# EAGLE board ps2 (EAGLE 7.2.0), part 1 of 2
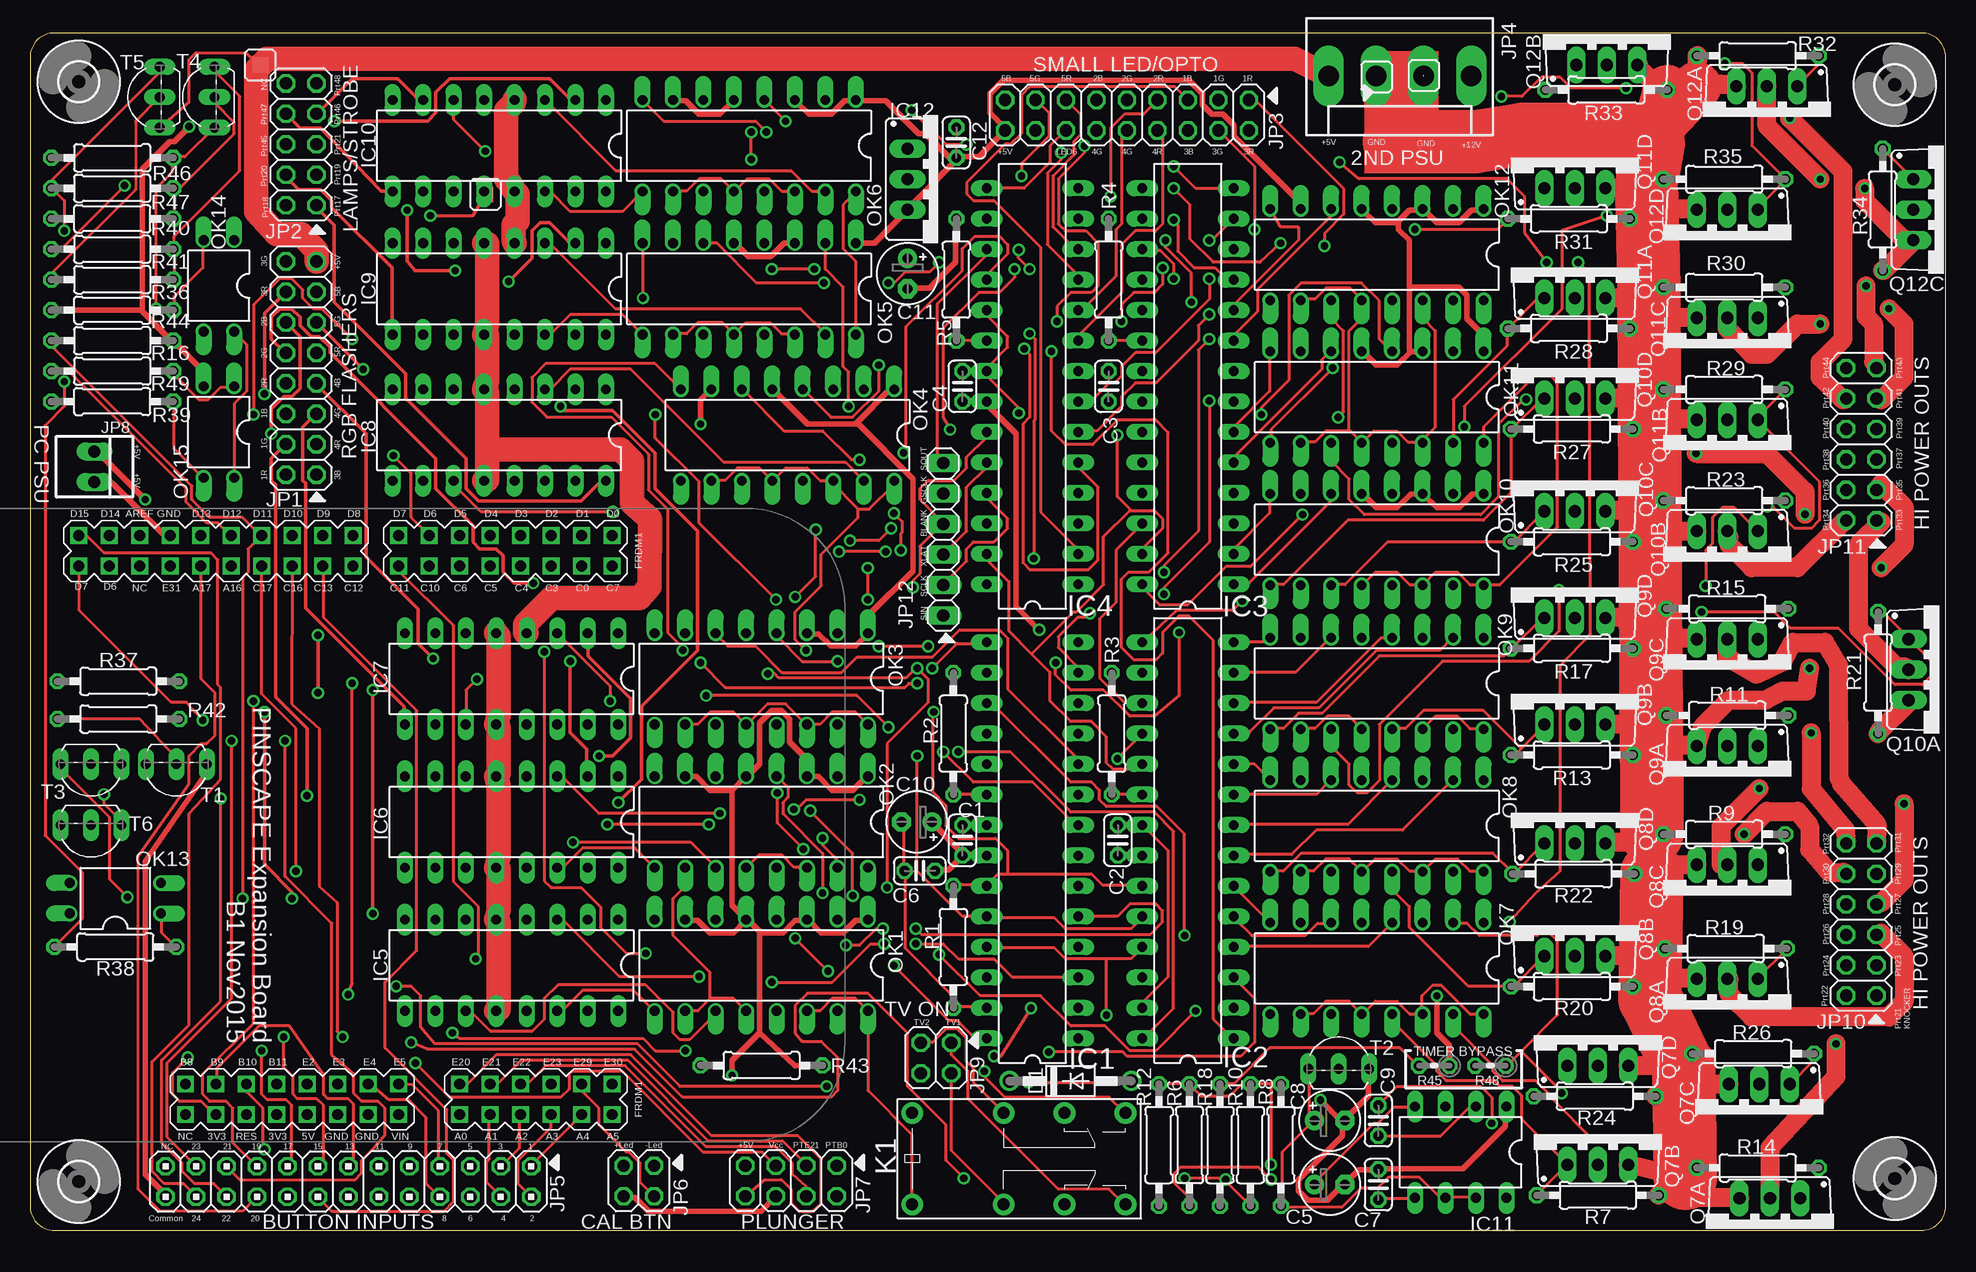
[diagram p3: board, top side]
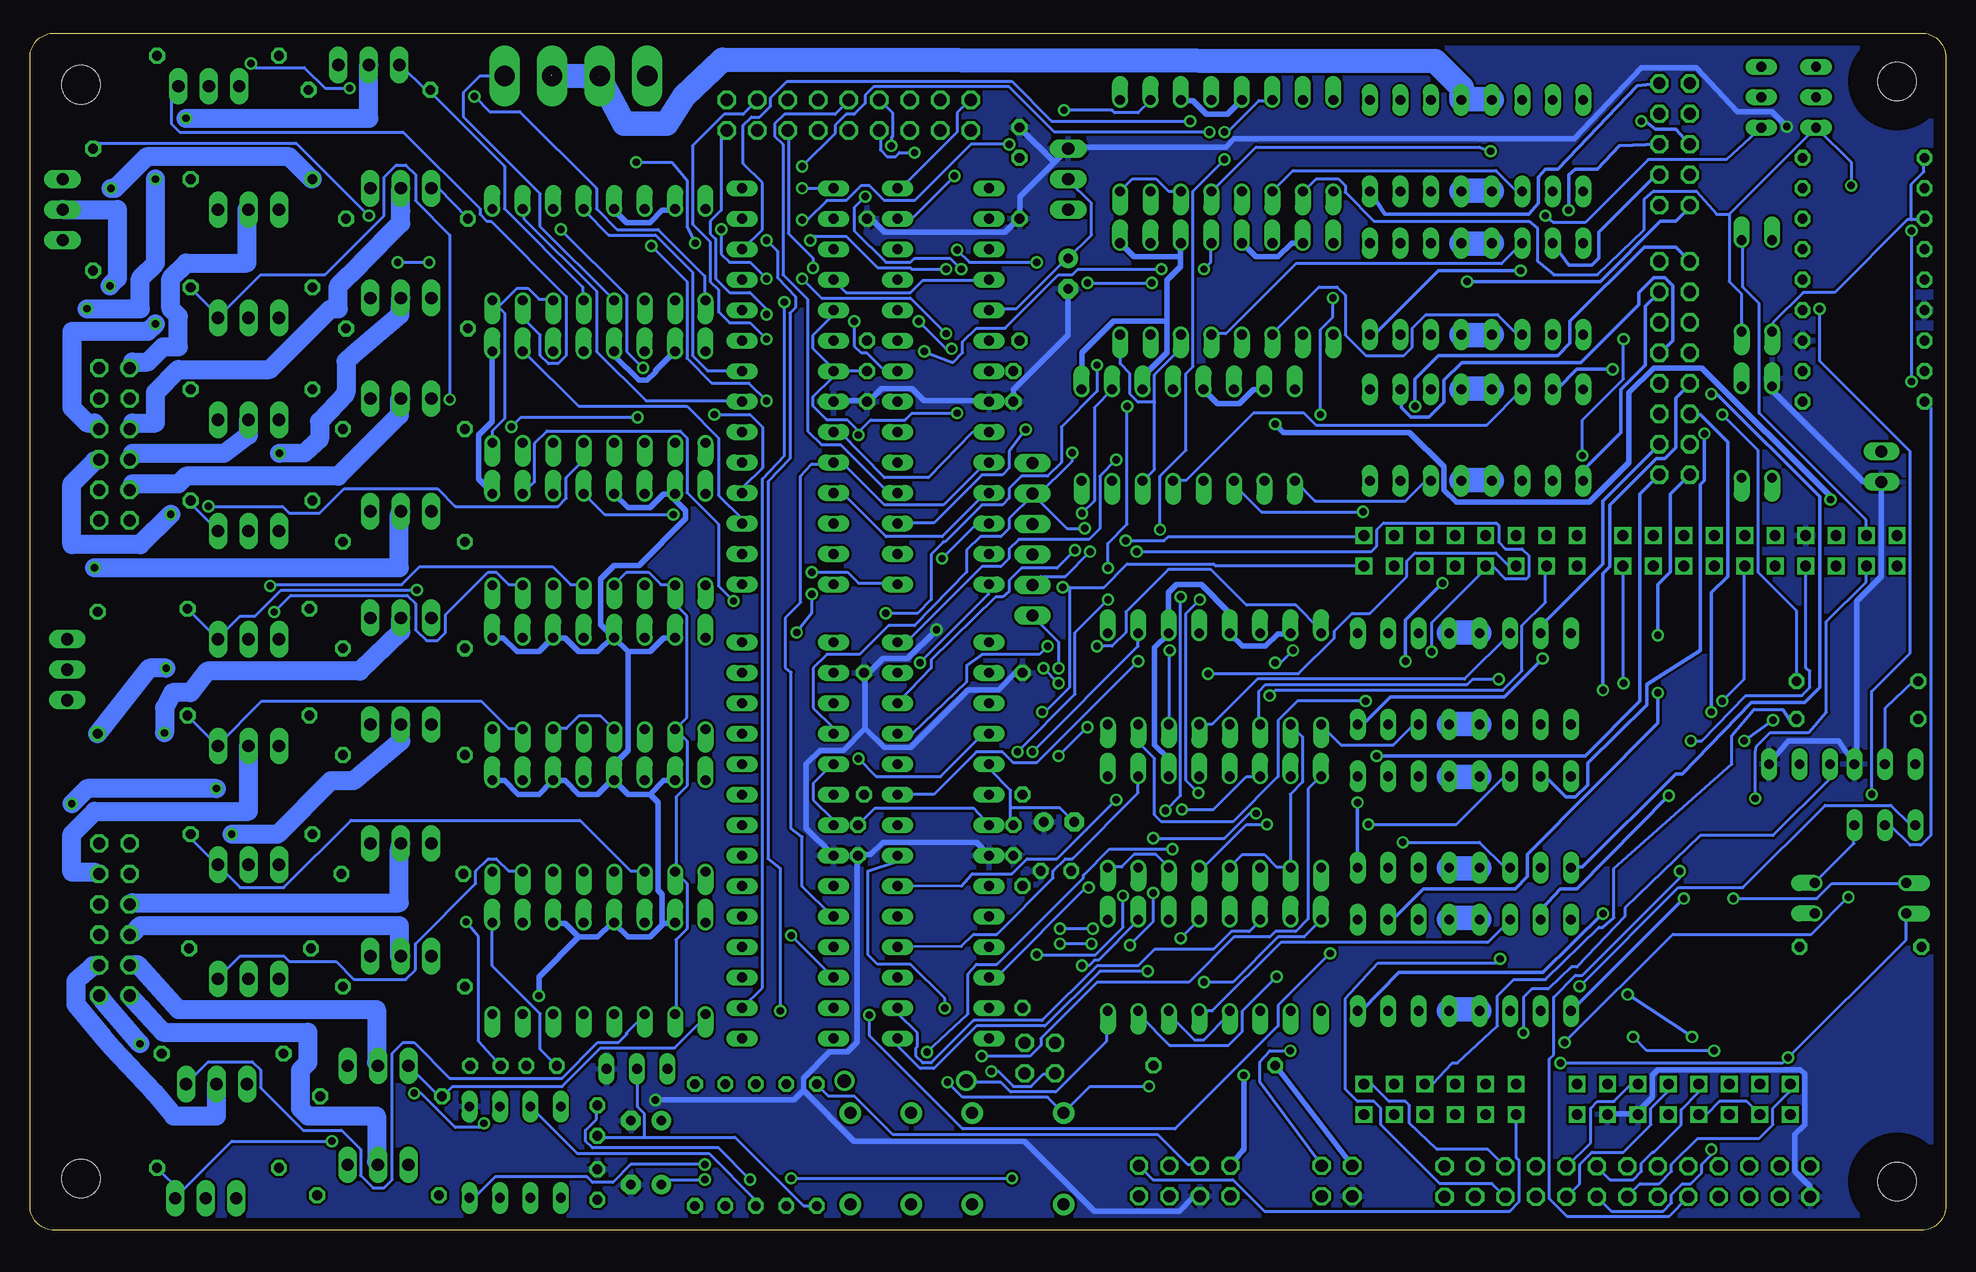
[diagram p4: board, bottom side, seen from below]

Size 159.69 x 99.81 mm. Coordinates in mm from the lower left corner, seen from the top.
Outline: 0,97.78 0,2.03 arc90 2.03,0 157.66,0 arc90 159.69,2.03 159.69,97.78 arc90 157.66,99.81 2.03,99.81 arc90 0,97.78
Copper layers (1*16): Top 0.035mm / dielectric 1.5mm / Bottom 0.035mm
Design rules "default": minimum track width 10mil, minimum drill 24mil, track to track 8mil, track to pad 8mil, pad to pad 8mil, via to via 8mil, smd to smd 8mil, copper to edge 40mil, drill to drill 8mil, minimum pad ring 10mil, minimum via ring 8mil, stop-mask expansion 4mil, vias tented up to drill 0mil, thermal gap 10mil
Net classes: 1 MOSFET Power & Ground: width 1.575 mm; 2 Lamps: width 0.305 mm; 3 Lamp Power & Ground: width 2.032 mm; 4 +5V: width 0.457 mm; 5 GND: width 0.457 mm

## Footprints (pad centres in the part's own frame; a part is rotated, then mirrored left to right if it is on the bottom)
C025-024X044 = drill 0.813 octagon: 1 -1.27,0; 2 1.27,0
E2,5-5 = drill 0.813 pad 1.6: + -1.27,0 | drill 0.813 pad 1.6 octagon: - 1.27,0
DO41-10 = drill 1.118: A 5.08,0; C -5.08,0
FRDM_KL25Z_NORMAL = drill 0.9 square: 3V3 24.13,-15.24; 5V 24.13,-7.62; A0 24.13,5.08; A1 24.13,7.62; A2 24.13,10.16; A3 24.13,12.7; A4 24.13,15.24; A5 24.13,17.78; AREF -24.13,-21.59; D0 -24.13,17.78; D1 -24.13,15.24; D2 -24.13,12.7; D3 -24.13,10.16; D4 -24.13,7.62; D5 -24.13,5.08; D6 -24.13,2.54; D7 -24.13,0; D8 -24.13,-3.81; D9 -24.13,-6.35; D10 -24.13,-8.89; D11 -24.13,-11.43; D12 -24.13,-13.97; D13 -24.13,-16.51; D14 -24.13,-24.13; D15 -24.13,-26.67; GND0 24.13,-2.54; GND1 24.13,-5.08; GND2 -24.13,-19.05; NC1 24.13,-17.78; NC2 -21.59,-21.59; P3V3 24.13,-10.16; PTA16 -21.59,-13.97; PTA17 -21.59,-16.51; PTB8 21.59,-17.78; PTB9 21.59,-15.24; PTB10 21.59,-12.7; PTB11 21.59,-10.16; PTC0 -21.59,15.24; PTC3 -21.59,12.7; PTC4 -21.59,10.16; PTC5 -21.59,7.62; PTC6 -21.59,5.08; PTC7 -21.59,17.78; PTC10 -21.59,2.54; PTC11 -21.59,0; PTC12 -21.59,-3.81; PTC13 -21.59,-6.35; PTC16 -21.59,-8.89; PTC17 -21.59,-11.43; PTD6 -21.59,-24.13; PTD7 -21.59,-26.67; PTE2 21.59,-7.62; PTE3 21.59,-5.08; PTE4 21.59,-2.54; PTE5 21.59,0; PTE20 21.59,5.08; PTE21 21.59,7.62; PTE22 21.59,10.16; PTE23 21.59,12.7; PTE29 21.59,15.24; PTE30 21.59,17.78; PTE31 -21.59,-19.05; RESET 24.13,-12.7; VIN 24.13,0
DIP28 = drill 0.813 long: 1 -15.24,-3.81; 2 -12.7,-3.81; 3 -10.16,-3.81; 4 -7.62,-3.81; 5 -5.08,-3.81; 6 -2.54,-3.81; 7 0,-3.81; 8 2.54,-3.81; 9 5.08,-3.81; 10 7.62,-3.81; 11 10.16,-3.81; 12 12.7,-3.81; 13 15.24,-3.81; 14 17.78,-3.81; 15 17.78,3.81; 16 15.24,3.81; 17 12.7,3.81; 18 10.16,3.81; 19 7.62,3.81; 20 5.08,3.81; 21 2.54,3.81; 22 0,3.81; 23 -2.54,3.81; 24 -5.08,3.81; 25 -7.62,3.81; 26 -10.16,3.81; 27 -12.7,3.81; 28 -15.24,3.81
DIL16 = drill 0.813 long: 1 -8.89,-3.81; 2 -6.35,-3.81; 3 -3.81,-3.81; 4 -1.27,-3.81; 5 1.27,-3.81; 6 3.81,-3.81; 7 6.35,-3.81; 8 8.89,-3.81; 9 8.89,3.81; 10 6.35,3.81; 11 3.81,3.81; 12 1.27,3.81; 13 -1.27,3.81; 14 -3.81,3.81; 15 -6.35,3.81; 16 -8.89,3.81
DIL08 = drill 0.813 long: 1 -3.81,-3.81; 2 -1.27,-3.81; 3 1.27,-3.81; 4 3.81,-3.81; 5 3.81,3.81; 6 1.27,3.81; 7 -1.27,3.81; 8 -3.81,3.81
TO220S = drill 1.016 long: 1 -2.54,-2.54; 2 0,-2.54; 3 2.54,-2.54
2X08 = drill 1.016 octagon: 1 -8.89,-1.27; 2 -8.89,1.27; 3 -6.35,-1.27; 4 -6.35,1.27; 5 -3.81,-1.27; 6 -3.81,1.27; 7 -1.27,-1.27; 8 -1.27,1.27; 9 1.27,-1.27; 10 1.27,1.27; 11 3.81,-1.27; 12 3.81,1.27; 13 6.35,-1.27; 14 6.35,1.27; 15 8.89,-1.27; 16 8.89,1.27
2X05 = drill 1.016 octagon: 1 -5.08,-1.27; 2 -5.08,1.27; 3 -2.54,-1.27; 4 -2.54,1.27; 5 0,-1.27; 6 0,1.27; 7 2.54,-1.27; 8 2.54,1.27; 9 5.08,-1.27; 10 5.08,1.27
2X09 = drill 1.016 octagon: 1 -10.16,-1.27; 2 -10.16,1.27; 3 -7.62,-1.27; 4 -7.62,1.27; 5 -5.08,-1.27; 6 -5.08,1.27; 7 -2.54,-1.27; 8 -2.54,1.27; 9 0,-1.27; 10 0,1.27; 11 2.54,-1.27; 12 2.54,1.27; 13 5.08,-1.27; 14 5.08,1.27; 15 7.62,-1.27; 16 7.62,1.27; 17 10.16,-1.27; 18 10.16,1.27
KK-156-4 = drill 1.7 pad 2.184 long: 1 -5.94,0; 2 -1.98,0; 3 1.98,0; 4 5.94,0
2X13 = drill 1.016 octagon: 1 -15.24,-1.27; 2 -15.24,1.27; 3 -12.7,-1.27; 4 -12.7,1.27; 5 -10.16,-1.27; 6 -10.16,1.27; 7 -7.62,-1.27; 8 -7.62,1.27; 9 -5.08,-1.27; 10 -5.08,1.27; 11 -2.54,-1.27; 12 -2.54,1.27; 13 0,-1.27; 14 0,1.27; 15 2.54,-1.27; 16 2.54,1.27; 17 5.08,-1.27; 18 5.08,1.27; 19 7.62,-1.27; 20 7.62,1.27; 21 10.16,-1.27; 22 10.16,1.27; 23 12.7,-1.27; 24 12.7,1.27; 25 15.24,-1.27; 26 15.24,1.27
2X02 = drill 1.016 octagon: 1 -1.27,-1.27; 2 -1.27,1.27; 3 1.27,-1.27; 4 1.27,1.27
2X04 = drill 1.016 octagon: 1 -3.81,-1.27; 2 -3.81,1.27; 3 -1.27,-1.27; 4 -1.27,1.27; 5 1.27,-1.27; 6 1.27,1.27; 7 3.81,-1.27; 8 3.81,1.27
22-23-2021 = drill 1 long: 1 -1.27,0; 2 1.27,0
2X06 = drill 1.016 octagon: 1 -6.35,-1.27; 2 -6.35,1.27; 3 -3.81,-1.27; 4 -3.81,1.27; 5 -1.27,-1.27; 6 -1.27,1.27; 7 1.27,-1.27; 8 1.27,1.27; 9 3.81,-1.27; 10 3.81,1.27; 11 6.35,-1.27; 12 6.35,1.27
1X06 = drill 1.016 long: 1 -6.35,0; 2 -3.81,0; 3 -1.27,0; 4 1.27,0; 5 3.81,0; 6 6.35,0
G5V-2 = drill 1 pad 1.8: 1 -8.89,-3.81; 4 -1.27,-3.81; 6 3.81,-3.81; 8 8.89,-3.81; 9 8.89,3.81; 11 3.81,3.81; 13 -1.27,3.81; 16 -8.89,3.81
DIL16' = drill 0.813 offset: 1 -8.89,-3.81; 2 -6.35,-3.81; 3 -3.81,-3.81; 4 -1.27,-3.81; 5 1.27,-3.81; 6 3.81,-3.81; 7 6.35,-3.81; 8 8.89,-3.81; 9 8.89,3.81; 10 6.35,3.81; 11 3.81,3.81; 12 1.27,3.81; 13 -1.27,3.81; 14 -3.81,3.81; 15 -6.35,3.81; 16 -8.89,3.81
DIL04 = drill 0.813 offset: 1 -1.27,-3.81; 2 1.27,-3.81; 3 1.27,3.81; 4 -1.27,3.81
TO220BV = drill 1.016 long: 1 -2.54,-2.54; 2 0,-2.54; 3 2.54,-2.54
0207/10 = drill 0.813 octagon: 1 -5.08,0; 2 5.08,0
0204V = drill 0.813 octagon: 1 -1.27,0; 2 1.27,0
TO92-EBC = drill 0.813 long: B 0,-1.27; C 2.54,-1.27; E -2.54,-1.27
JP0 = smd 1.27 x 1.27: P$1 0,1.27; P$2 0,1.27
3,2 = hole 3.2: 0,0

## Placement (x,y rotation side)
C1  100nF  [C025-024X044]  77.72,32.51 90 top
C2  100nF  [C025-024X044]  90.68,32.51 90 top
C3  100nF  [C025-024X044]  89.92,70.36 90 top
C4  100nF  [C025-024X044]  77.72,70.36 90 top
C5  1uF  [E2,5-5]  108.33,3.81 0 top
C6  4.7uF  [C025-024X044]  74.17,29.97 180 top
C7  100nF  [C025-024X044]  112.39,3.81 90 top
C8  1uF  [E2,5-5]  108.33,9.14 0 top
C9  100nF  [C025-024X044]  112.39,9.14 90 top
C10  100uF  [E2,5-5]  73.91,34.04 180 top
C11  100uF  [E2,5-5]  73.15,79.76 270 top
C12  100nF  [C025-024X044]  77.22,90.68 90 top
D1  1N4007  [DO41-10]  86.73,12.45 0 top
FRDM1  KL25Z  [FRDM_KL25Z_NORMAL]  30.73,33.78 270 top
IC1  TLC5940NT  [DIP28]  83.57,31.24 90 top
IC2  TLC5940NT  [DIP28]  96.52,31.24 90 top
IC3  TLC5940NT  [DIP28]  96.52,69.09 90 top
IC4  TLC5940NT  [DIP28]  83.57,69.09 90 top
IC5  ULN2064BN  [DIL16]  40.13,22.1 180 top
IC6  ULN2064BN  [DIL16]  40.13,34.04 180 top
IC7  ULN2064BN  [DIL16]  40.13,45.97 180 top
IC8  ULN2064BN  [DIL16]  39.12,66.29 180 top
IC9  ULN2064BN  [DIL16]  39.12,78.49 180 top
IC10  ULN2064BN  [DIL16]  39.12,90.42 180 top
IC11  ICM7555  [DIL08]  119.25,6.52 180 top
IC12  LD1117AV33  [TO220S]  75.69,87.63 270 top
JP1  M20-9760846  [2X08]  22.61,71.88 90 top
JP2  M20-9760546  [2X05]  22.61,90.54 90 top
JP3  M20-9760746  [2X09]  91.44,92.96 180 top
JP4  KK-156-4  [KK-156-4]  114.19,96.24 180 top
JP5  M20-9761346  [2X13]  26.54,4.06 180 top
JP6  M20-9760246  [2X02]  50.75,4.11 180 top
JP7  M20-9760446  [2X04]  63.44,4.11 180 top
JP8  22-23-2021  [22-23-2021]  5.37,63.67 270 top
JP9  M20-9760246  [2X02]  75.51,14.36 180 top
JP10  M20-9760646  [2X06]  152.65,25.91 90 top
JP11  M20-9760646  [2X06]  152.65,65.53 90 top
JP12  M20-9990646  [1X06]  76.12,57.61 90 top
K1  G5V-2  [G5V-2]  82.42,5.97 0 top
OK1  PC847  [DIL16']  60.96,22.1 180 top
OK2  PC847  [DIL16']  60.96,34.04 180 top
OK3  PC847  [DIL16']  60.96,45.97 180 top
OK4  PC847  [DIL16']  63.14,66.29 180 top
OK5  PC847  [DIL16']  59.94,78.49 180 top
OK6  PC847  [DIL16']  59.94,90.42 180 top
OK7  PC847  [DIL16']  112.27,21.84 180 top
OK8  PC847  [DIL16']  112.27,33.72 180 top
OK9  PC847  [DIL16']  112.27,45.59 180 top
OK10  PC847  [DIL16']  112.27,57.58 180 top
OK11  PC847  [DIL16']  112.27,69.46 180 top
OK12  PC847  [DIL16']  112.27,81.33 180 top
OK13  PC817  [DIL04]  7.11,27.69 90 top
OK14  PC817  [DIL04]  15.75,78.74 180 top
OK15  PC817  [DIL04]  15.75,66.55 180 top
Q7A  BUK7575-55A  [TO220BV]  145.03,0.13 180 top
Q7B  BUK7575-55A  [TO220BV]  130.68,8 0 top
Q7C  BUK7575-55A  [TO220BV]  144.15,9.65 180 top
Q7D  BUK7575-55A  [TO220BV]  130.68,16.26 0 top
Q8A  BUK7575-55A  [TO220BV]  141.48,18.41 180 top
Q8B  BUK7575-55A  [TO220BV]  128.78,25.4 0 top
Q8C  BUK7575-55A  [TO220BV]  141.48,27.94 180 top
Q8D  BUK7575-55A  [TO220BV]  128.78,34.8 0 top
Q9A  BUK7575-55A  [TO220BV]  141.48,37.85 180 top
Q9B  BUK7575-55A  [TO220BV]  128.78,44.7 0 top
Q9C  BUK7575-55A  [TO220BV]  141.48,46.74 180 top
Q9D  BUK7575-55A  [TO220BV]  128.78,53.59 0 top
Q10A  BUK7575-55A  [TO220BV]  159.13,46.74 270 top
Q10B  BUK7575-55A  [TO220BV]  141.48,55.75 180 top
Q10C  BUK7575-55A  [TO220BV]  128.78,62.48 0 top
Q10D  BUK7575-55A  [TO220BV]  128.78,71.88 0 top
Q11A  BUK7575-55A  [TO220BV]  128.78,80.26 0 top
Q11B  BUK7575-55A  [TO220BV]  141.48,65.02 180 top
Q11C  BUK7575-55A  [TO220BV]  141.48,73.53 180 top
Q11D  BUK7575-55A  [TO220BV]  128.78,89.41 0 top
Q12A  BUK7575-55A  [TO220BV]  144.78,92.84 180 top
Q12B  BUK7575-55A  [TO220BV]  131.44,99.69 0 top
Q12C  BUK7575-55A  [TO220BV]  159.51,85.09 270 top
Q12D  BUK7575-55A  [TO220BV]  141.48,82.55 180 top
R1  10K  [0207/10]  76.96,23.62 270 top
R2  4K  [0207/10]  76.96,41.4 90 top
R3  4K  [0207/10]  90.17,41.4 90 top
R4  4K  [0207/10]  89.92,79.25 90 top
R5  2.2K  [0207/10]  77.22,79.25 90 top
R6  1M  [0207/10]  96.65,7.11 90 top
R7  1K  [0207/10]  130.68,2.92 180 top
R8  2.2M  [0207/10]  104.27,7.11 270 top
R9  1K  [0207/10]  141.22,33.02 0 top
R10  100K  [0207/10]  101.73,7.11 270 top
R11  1K  [0207/10]  141.48,42.93 0 top
R12  100K  [0207/10]  94.11,7.11 270 top
R13  1K  [0207/10]  128.52,39.62 180 top
R14  1K  [0207/10]  144.02,5.21 0 top
R15  1K  [0207/10]  141.48,51.82 0 top
R16  10K  [0207/10]  6.86,74.17 180 top
R17  1K  [0207/10]  128.52,48.51 180 top
R18  47R  [0207/10]  99.19,7.11 270 top
R19  1K  [0207/10]  141.35,23.5 0 top
R20  1K  [0207/10]  128.52,20.32 180 top
R21  1K  [0207/10]  154.05,46.48 90 top
R22  1K  [0207/10]  128.65,29.72 180 top
R23  1K  [0207/10]  141.22,60.83 0 top
R24  1K  [0207/10]  130.43,11.18 180 top
R25  1K  [0207/10]  128.52,57.4 180 top
R26  1K  [0207/10]  143.64,14.73 0 top
R27  1K  [0207/10]  128.52,66.8 180 top
R28  1K  [0207/10]  128.27,75.18 180 top
R29  1K  [0207/10]  141.22,70.1 0 top
R30  1K  [0207/10]  141.22,78.61 0 top
R31  1K  [0207/10]  128.27,84.33 180 top
R32  1K  [0207/10]  144.02,97.92 0 top
R33  1K  [0207/10]  131.39,95.07 180 top
R34  1K  [0207/10]  154.43,85.09 90 top
R35  1K  [0207/10]  141.22,87.63 0 top
R36  560R  [0207/10]  6.86,76.71 0 top
R37  2.2K  [0207/10]  7.37,45.77 180 top
R38  220R  [0207/10]  7.11,23.62 0 top
R39  560R  [0207/10]  6.86,71.63 180 top
R40  10K  [0207/10]  6.86,84.33 0 top
R41  4.7K  [0207/10]  6.86,81.79 180 top
R42  2.2K  [0207/10]  7.37,42.62 180 top
R43  82R  [0207/10]  60.97,13.74 180 top
R44  4.7K  [0207/10]  6.86,79.25 180 top
R45  0R  [0204V]  117.04,13.72 180 top
R46  10K  [0207/10]  6.86,89.41 180 top
R47  22K  [0207/10]  6.86,86.87 180 top
R48  0R  [0204V]  121.73,13.72 180 top
R49  2.2K  [0207/10]  6.86,69.09 0 top
T1  2N4401  [TO92-EBC]  12.19,37.59 180 top
T2  2N4403  [TO92-EBC]  109.09,14.73 0 top
T3  2N4401  [TO92-EBC]  5.08,37.59 180 top
T4  2N4401  [TO92-EBC]  14.11,94.46 90 top
T5  2N4403  [TO92-EBC]  9.54,94.46 90 top
T6  2N4401  [TO92-EBC]  5.08,32.51 180 top
U$1  NETJUMPER  [JP0]  19.2,98.41 180 top
U$2  NETJUMPER  [JP0]  116.19,97.55 180 top
U$3  NETJUMPER  [JP0]  37.97,85.09 0 top
U$4  NETJUMPER  [JP0]  112.24,94.89 0 top
U$16  [3,2]  4.06,95.76 270 top
U$17  [3,2]  155.45,4.32 90 top
U$18  [3,2]  4.06,4.06 0 top
U$19  [3,2]  155.45,95.5 0 top

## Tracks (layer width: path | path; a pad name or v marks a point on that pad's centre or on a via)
3V3_KL25Z  (via drill 0.61)
  Top 0.254: v13.14,14.4 11.89,13.14 11.89,11.32 12.46,10.74 14.29,10.74 15.43,9.6 FRDM1.3V3 | 103.44,12.23 104.24,12.23 R8.1 | 103.44,12.23 101.73,12.23 R10.1 101.61,12.23 101.04,12.23 100.01,11.2 97.61,11.2 96.7,12.12 R6.2 96.58,12.23 94.18,12.23 R12.1 | 103.44,12.23 v103.44,5.49 | v32.12,13.95 34.98,11.09 44.23,11.09 44.92,11.77 44.92,13.03 45.15,13.26 49.38,13.26 56.12,6.51 61.04,6.51 JP7.5
  Bottom 0.254: OK13.4 3.31,26.4 3.31,24.23 v13.14,14.4 13.6,13.95 v32.12,13.95 | FRDM1.P3V3 20.57,9.72 19.89,9.72 18.86,10.74 16.57,10.74 15.54,9.72 FRDM1.3V3 | v103.44,5.49 109.61,5.49 111.1,4 112.81,4 113.27,4.46 120.93,4.46 122.64,2.74 122.99,2.74 IC11.8 | JP7.5 62.18,5.49 63.21,5.49 65.72,8 87.78,8 90.98,11.2 93.15,11.2 94.07,12.12 R12.1
+5V  (via drill 0.61)
  Top 0.457: OK10.5 111.1,61.38 112.24,60.24 113.96,60.24 115.1,61.38 116.01,61.38 OK10.3 116.24,61.27 117.27,60.24 119.1,60.24 120.24,61.38 121.16,61.38 OK10.1 | 115.1,73.27 OK11.3 | 115.1,73.27 113.96,72.12 112.24,72.12 111.1,73.27 OK11.5 | 113.96,84.01 114.99,85.04 116.01,85.04 OK12.3 116.24,85.04 117.27,84.01 119.1,84.01 120.13,85.04 121.16,85.04 OK12.1 | 113.96,84.01 112.13,84.01 OK12.5 | 114.99,78.64 114.99,82.53 114.07,83.44 114.07,83.9 113.96,84.01 | 114.99,78.64 114.99,73.38 115.1,73.27 | OK11.1 121.16,74.64 119.79,76.01 119.79,77.95 119.1,78.64 114.99,78.64 | v117.27,19.55 117.27,16.46 118.3,15.43 R45.1 | OK2.1 69.84,37.95 68.58,36.69 66.86,36.69 65.72,37.83 64.81,37.83 OK2.3 64.69,38.06 64.69,39.32 63.32,40.69 63.32,42.63 62.64,43.32 61.84,43.32 60.81,42.29 60.81,38.86 59.89,37.95 OK2.5 59.66,37.83 58.52,36.69 | OK3.3 64.81,49.72 65.72,49.72 66.75,48.69 68.81,48.69 69.84,49.72 OK3.1 69.95,49.95 69.95,51.32 73.61,54.98 73.61,62.64 68.92,67.32 | 58.52,36.69 56.69,36.69 55.55,37.83 54.63,37.83 OK2.7 | OK1.7 54.63,25.83 55.66,25.83 56.69,24.8 58.64,24.8 59.66,25.83 OK1.5 | 60.92,24.8 62.75,24.8 63.78,25.83 64.69,25.83 OK1.3 64.92,25.83 65.95,24.8 67.78,24.8 68.81,25.83 69.84,25.83 OK1.1 | 60.92,24.8 59.89,25.83 OK1.5 | 58.52,36.69 58.52,27.09 59.55,26.06 OK1.5 | v58.52,12.92 58.52,14.17 60.81,16.46 | 60.81,16.46 60.81,24.69 60.92,24.8 | OK5.3 62.87,82.3 61.72,81.15 59.89,81.15 58.75,82.3 OK5.5 | OK6.7 53.61,94.18 54.63,94.18 55.78,93.04 57.49,93.04 58.64,94.18 OK6.5 | OK6.3 63.78,94.18 64.92,93.04 66.75,93.04 67.89,94.18 68.81,94.18 OK6.1 69.04,94.18 71.32,94.18 74.07,91.44 74.64,91.44 76.81,89.27 C12.1
  Top 0.457: C12.1 77.27,89.5 79.1,89.5 81.27,91.67 JP3.18 81.27,91.9 80.01,93.15 80.01,94.75 81.15,95.9 96.58,95.9 97.73,94.75 97.73,93.84 98.53,93.04 99.44,93.04 100.36,92.13 100.36,91.21 105.84,85.72 105.84,85.15 OK12.7 | OK5.1 70.41,82.3 73.15,85.04 IC12.3 73.27,85.27 77.04,89.04 77.04,89.27 C12.1 | v9.6,60.92 5.6,64.92 5.37,64.92 JP8.1 | v55.89,67.21 55.89,69.27 56.69,70.07 OK4.7 | 68.92,67.32 68.81,67.21 64.81,67.21 61.95,70.07 OK4.5 | 68.92,67.32 71.67,70.07 72.01,70.07 OK4.1 | 60.81,16.46 63.78,13.72 R43.1
  Bottom 0.457: OK10.5 109.84,60.24 108.01,60.24 106.87,61.38 105.96,61.38 OK10.7 105.96,61.15 105.96,60.92 105.04,60.01 105.04,59.32 108.93,55.44 110.98,55.44 112.13,54.29 112.13,50.52 111.21,49.61 OK9.5 | OK11.1 121.16,67.44 122.3,66.29 122.3,62.64 121.16,61.49 OK10.1 | OK11.7 105.96,73.27 107.56,71.67 107.56,71.55 108.24,70.87 108.93,70.87 110.98,72.92 110.98,73.27 OK11.5 | OK12.7 105.96,85.04 106.98,85.04 108.01,84.01 109.96,84.01 110.98,85.04 OK12.5 | 106.87,25.6 105.96,25.6 OK7.7 | 106.87,25.6 108.01,24.46 109.84,24.46 110.98,25.6 OK7.5 111.21,25.6 112.36,24.46 113.96,24.46 | 113.96,24.46 115.1,25.6 116.01,25.6 OK7.3 | v117.27,19.55 117.27,21.14 113.96,24.46 | 108.01,36.35 106.87,37.49 105.96,37.49 OK8.7 | 108.01,36.35 109.84,36.35 110.98,37.49 OK8.5 | OK8.5 111.21,37.49 112.36,36.35 113.96,36.35 115.1,37.49 116.01,37.49 OK8.3 116.24,37.38 117.27,36.35 118.99,36.35 120.13,37.49 121.16,37.49 OK8.1 | 109.84,48.23 108.01,48.23 106.87,49.38 105.96,49.38 OK9.7 | 109.84,48.23 110.98,49.38 OK9.5 | OK9.5 111.21,49.38 112.36,48.23 113.96,48.23 115.1,49.38 116.01,49.38 OK9.3 116.24,49.26 117.27,48.23 119.1,48.23 120.24,49.38 121.16,49.38 OK9.1 | 109.84,48.23 109.84,40.01 110.87,38.98 110.87,37.72 OK8.5 | 108.01,36.35 107.33,35.66 107.33,28.35 106.98,28 106.98,25.72 106.87,25.6 | OK3.7 54.63,49.72 55.66,49.72 56.69,48.69 58.64,48.69 59.66,49.72 OK3.5 59.78,49.95 59.78,51.55 62.06,53.84 64.12,53.84 64.81,53.15 64.81,49.95 OK3.3 64.81,49.72 65.95,48.58 65.95,40.46 64.81,39.32 64.81,37.95 OK2.3 | JP7.7 59.55,5.49 58.64,6.63 58.52,6.74 v58.52,12.92 | OK5.7 54.52,82.3 55.66,81.15 57.49,81.15 58.64,82.3 OK5.5
  Bottom 0.457: 64.92,75.78 64.92,79.21 63.78,80.35 63.78,81.15 | 64.92,75.78 64.92,73.15 66.86,71.21 66.86,70.18 OK4.3 | 63.78,81.15 63.78,82.3 OK5.3 | 64.92,75.78 69.38,75.78 72.01,73.15 72.01,70.18 OK4.1 | OK6.3 63.66,94.18 62.75,94.18 61.61,93.04 59.89,93.04 58.75,94.18 OK6.5 | 63.78,81.15 67.67,81.15 68.81,82.3 OK5.1 | OK4.5 60.69,68.92 58.86,68.92 57.72,70.07 56.81,70.07 OK4.7 | v9.6,60.92 9.6,61.15 20.34,71.89 24.35,71.89 26.4,69.84 26.4,64.01 29.72,60.69 40.8,60.69 41.83,61.72 41.83,63.66 44.69,66.52 55.21,66.52 v55.89,67.21
+5V_PSU2  (via drill 0.61)
  Top 0.254: OK15.4 17.03,68.92 18.06,69.95 18.06,73.84 17.03,74.87 OK14.4 | v7.89,87.1 2.63,81.84 1.83,81.84 R41.2 | OK6.10 53.61,86.64 54.75,86.64 55.78,87.67 57.61,87.67 58.64,86.64 OK6.12 58.75,86.64 59.78,87.67 61.61,87.67 62.64,86.64 63.66,86.64 OK6.14 | OK5.16 68.81,74.75 68.81,80.81 67.78,81.84 67.78,85.5 68.81,86.53 OK6.16 | OK5.10 53.61,74.75 54.75,74.75 55.66,75.67 57.72,75.67 58.64,74.75 OK5.12 59.66,75.67 61.72,75.67 62.64,74.75 63.66,74.75 OK5.14 | OK4.10 56.81,62.52 57.95,62.52 58.98,63.55 60.81,63.55 OK4.12 61.95,62.52 62.98,63.55 64.81,63.55 65.84,62.52 66.86,62.52 OK4.14 66.75,62.41 69.04,60.12 | 69.04,60.12 69.95,60.12 72.01,62.18 72.01,62.41 OK4.16 | OK2.14 64.69,30.29 63.66,30.29 62.64,31.32 60.81,31.32 59.78,30.29 OK2.12 | OK3.10 54.63,42.18 55.66,42.18 56.69,43.2 58.64,43.2 59.66,42.18 OK3.12 59.78,42.18 61.49,43.89 62.98,43.89 64.69,42.18 OK3.14 64.81,42.18 65.84,42.18 66.86,43.2 68.81,43.2 OK3.16 | OK1.10 55.66,18.29 56.69,19.32 | 56.69,19.32 58.64,19.32 59.66,18.29 OK1.12 | OK1.14 65.84,18.29 66.86,19.32 68.81,19.32 69.84,18.29 OK1.16 69.84,18.17 69.84,11.66 73.5,8 73.5,2.17 K1.1 | 56.69,19.32 56.69,21.49 53.61,24.57 53.61,27.66 54.52,28.57 54.52,30.18 OK2.10 | 69.04,60.12 69.04,59.44 65.95,56.35 65.95,53.72 63.78,51.55 63.78,49.26 v64.69,48.35 | U$1.P$2 17.95,98.18 13.83,98.18 13.26,97.61 13.26,94.07 T5.E
  Bottom 0.254: v7.89,87.1 7.89,89.04 10.74,91.9 T5.E 10.86,91.9 18.06,84.7 | 18.06,84.7 18.06,79.1 17.03,78.07 17.03,74.98 OK14.4 | OK6.16 67.78,87.67 65.84,87.67 64.81,86.64 63.78,86.64 OK6.14 | 65.95,69.04 65.95,63.44 66.86,62.52 OK4.14 | 65.95,69.04 65.95,71.32 63.78,73.5 63.78,74.64 OK5.14 | 65.95,69.04 67.32,69.04 68.01,69.72 68.01,71.44 68.81,72.24 68.81,74.64 OK5.16 | OK2.12 59.66,30.29 58.64,31.32 56.81,31.32 55.78,30.29 54.63,30.29 OK2.10 54.63,30.4 54.63,36.35 53.61,37.38 53.61,41.15 54.52,42.06 OK3.10 | OK2.16 69.84,30.29 68.69,30.29 67.67,31.32 65.84,31.32 64.81,30.29 OK2.14 | D1.C 81.61,12.34 78.75,12.34 77.95,11.54 74.18,11.54 69.95,15.77 69.95,18.29 OK1.16 | OK1.12 59.78,18.29 59.78,17.95 61.84,15.89 62.64,15.89 64.69,17.95 64.69,18.29 OK1.14 | v64.69,48.35 64.69,42.18 OK3.14 | 18.06,84.7 19.09,84.7 20.8,86.64 24.35,86.64 25.15,85.95 25.15,83.44 29.03,79.67 32.69,79.67 34.06,80.81 34.06,83.55 34.75,84.12 47.66,84.12 50.06,86.53 50.06,87.1 50.63,87.67 52.46,87.67 53.49,86.64 OK6.10
+12V
  Top 0.254: OK12.10 105.96,77.61 107.1,77.61 108.01,78.52 110.07,78.52 110.98,77.61 OK12.12 110.98,77.5 110.98,76.01 109.96,74.98 109.96,66.64 | 109.96,66.64 110.07,66.64 110.98,65.72 OK11.12 111.1,65.72 112.01,66.64 113.96,66.64 114.87,65.72 116.01,65.72 OK11.14 116.01,65.84 117.16,66.98 117.16,74.98 116.13,76.01 116.13,77.5 OK12.14 | 109.96,66.64 108.01,66.64 107.1,65.72 105.96,65.72 OK11.10 | OK7.10 105.96,18.06 106.98,18.06 108.01,19.09 109.96,19.09 110.98,18.06 OK7.12 111.1,18.06 112.13,19.09 113.96,19.09 114.99,18.06 116.01,18.06 OK7.14 116.01,18.17 116.01,19.55 116.93,20.46 117.61,20.46 120.02,18.06 121.16,18.06 OK7.16 | OK10.12 111.1,53.84 112.13,54.86 113.96,54.86 114.99,53.84 116.01,53.84 OK10.14 116.13,53.84 117.16,54.86 118.99,54.86 120.02,53.84 121.16,53.84 OK10.16 121.27,53.84 122.53,53.84 127.33,58.64 127.33,70.64 126.76,71.21 125.39,71.21 121.16,66.98 OK11.16 | OK8.10 105.96,29.95 106.98,29.95 108.01,30.98 109.96,30.98 110.98,29.95 OK8.12 111.1,29.95 112.13,30.98 113.96,30.98 114.99,29.95 116.01,29.95 OK8.14 116.13,29.95 117.16,30.98 118.99,30.98 120.02,29.95 121.16,29.95 OK8.16 | OK9.10 105.96,41.83 107.1,41.83 108.13,42.86 109.96,42.86 110.98,41.83 OK9.12 | OK9.14 117.16,42.86 118.99,42.86 120.02,41.83 121.16,41.83 OK9.16
  Bottom 0.254: OK11.16 121.16,66.64 120.13,67.67 120.13,76.47 121.16,77.5 OK12.16 120.59,77.04 119.1,78.52 118.19,78.52 117.27,77.61 116.13,77.61 OK12.14 | JP4.1 122.19,96.24 123.56,94.87 123.56,92.81 117.16,86.41 117.16,83.67 111.1,77.61 OK12.12 | OK10.12 110.98,53.84 109.96,54.86 108.13,54.86 107.1,53.84 105.96,53.84 OK10.10 105.84,53.72 105.84,52.12 104.93,51.21 104.93,42.75 105.84,41.83 OK9.10 105.84,41.72 104.93,40.8 104.93,37.03 105.84,36.12 105.84,29.95 OK8.10 104.93,28.92 104.93,25.15 105.84,24.23 105.84,18.06 OK7.10 | OK9.14 116.01,41.83 114.99,41.83 113.96,42.86 112.13,42.86 111.1,41.83 OK9.12
ALT_MOSFETIN1  (via drill 0.61)
  Top 0.254: v123.33,25.72 125.5,28.12 127.56,29.95 127.56,47.09 130.07,49.72 129.96,74.3 129.96,79.78 v129.04,80.7 | v126.42,80.7 124.59,83.1 124.59,86.18 123.1,87.67 110.76,87.67 v109.16,89.04 | v104.24,82.3 102.53,80.7 98.64,80.7 96.7,82.64 96.7,85.5 v95.33,86.87
  Bottom 0.254: R48.2 122.3,15.77 122.3,24.46 v123.33,25.72 | v129.04,80.7 v126.42,80.7 | v109.16,89.04 106.19,89.04 104.93,87.55 104.93,83.67 v104.24,82.3 | v95.33,86.87 IC3.15
DARLINGTONIN1  (via drill 0.61)
  Top 0.254: IC1.28 78.75,16 77.27,17.49 76.58,17.49 v72.01,22.06
  Bottom 0.254: v72.01,22.06 71.44,22.06 70.98,22.52 70.64,22.52 67.32,25.83 OK1.2
DARLINGTONIN2  (via drill 0.61)
  Top 0.254: v63.78,24.35 v66.52,21.6
  Bottom 0.254: v66.52,21.6 70.52,21.6 75.09,17.03 80.81,17.03 84.35,13.49 85.5,13.49 87.33,15.32 87.33,16 IC1.1 | v63.78,24.35 62.29,25.83 OK1.4
DARLINGTONIN3
  Bottom 0.254: IC1.2 87.33,18.52 87.33,18.06 85.72,16.46 85.72,15.32 85.84,15.2 85.84,14.52 85.27,13.95 84.58,13.95 81.04,17.49 75.32,17.49 70.75,22.06 67.32,22.06 65.95,23.43 61.04,23.43 59.55,24.92 58.06,24.92 57.15,25.83 OK1.6
DARLINGTONIN4  (via drill 0.61)
  Top 0.254: v73.84,23.89 76.12,23.89 77.38,22.63 80.35,22.63 81.84,21.14 87.33,21.14 IC1.3 | v71.21,23.89 70.07,23.89 66.86,20.69 v61.84,20.69
  Bottom 0.254: v71.21,23.89 v73.84,23.89 | v61.84,20.69 59.44,20.69 55.66,24.46 53.49,24.46 52.12,25.83 OK1.8
DARLINGTONIN5
  Bottom 0.254: OK2.2 67.32,37.83 67.32,36.46 72.81,30.98 73.38,30.98 74.41,29.95 74.41,29.38 79.1,24.69 81.04,24.69 82.07,23.66 IC1.4
DARLINGTONIN6  (via drill 0.61)
  Top 0.254: v73.84,25.15 74.3,24.69 93.38,24.69 94.41,25.72 94.41,26.63 93.84,27.2 91.67,27.2 90.64,26.18 87.44,26.18 IC1.5 | v71.09,25.15 70.52,25.15 69.15,23.77 v68.01,23.77 | v66.06,28.12 66.06,31.43 62.75,34.75 62.75,35.66 63.21,36.12 63.21,36.92 62.29,37.83 OK2.4
  Bottom 0.254: v71.09,25.15 v73.84,25.15 | v68.01,23.77 66.06,25.72 v66.06,28.12
DARLINGTONIN7  (via drill 0.61)
  Top 0.254: v63.66,35.09 63.89,35.09 64.69,35.89 v69.15,35.89
  Bottom 0.254: v63.66,35.09 61.04,35.09 58.29,37.83 57.15,37.83 OK2.6 | v69.15,35.89 74.07,30.98 76.58,30.98 77.84,29.72 81.15,29.72 82.07,28.69 IC1.6
DARLINGTONIN8  (via drill 0.61)
  Top 0.254: v80.35,14.52 80.92,14.52 v83.44,18.52
  Bottom 0.254: v83.44,18.52 83.44,19.32 86.3,22.17 89.04,22.17 89.84,22.97 89.84,29.95 87.44,30.75 87.44,31.2 IC1.7 | v80.35,14.52 76.35,14.52 75.44,15.43 75.44,16 70.75,20.69 63.09,20.69 59.32,24.46 56.35,24.46 55.89,24.92 54.18,24.92 53.15,25.95 53.15,36.8 52.12,37.83 OK2.8
DARLINGTONIN9  (via drill 0.61)
  Top 0.254: v76.12,39.89 78.64,37.38 83.55,37.38 87.1,33.83 87.33,33.83 IC1.8
  Bottom 0.254: v76.12,39.89 67.32,48.69 67.32,49.72 OK3.2
DARLINGTONIN10  (via drill 0.61)
  Top 0.254: v67.32,47.43 64.35,47.43 62.29,49.49 62.29,49.72 OK3.4
  Bottom 0.254: v67.32,47.43 75.78,38.98 77.72,38.98 78.64,39.89 80.81,39.89 84.35,36.35 87.33,36.35 IC1.9
DARLINGTONIN11
  Top 0.254: IC1.10 87.33,38.86 87.33,39.32 81.5,45.15 81.5,49.38 80.81,50.06 77.5,50.06 75.21,47.78 68.92,47.78 67.67,46.52 62.64,46.52 60.47,48.69 58.18,48.69 57.15,49.72 OK3.6
DARLINGTONIN12  (via drill 0.61)
  Top 0.254: v70.75,48.69 v74.87,48.69
  Bottom 0.254: v74.87,48.69 75.55,48.01 80.35,48.01 81.61,47.09 81.61,45.72 86.18,41.38 IC1.11 | v70.75,48.69 69.49,48.69 68.35,49.84 68.35,51.55 64.81,55.09 61.27,55.09 58.29,52.12 54.18,52.12 52.12,50.06 52.12,49.84 OK3.8
DARLINGTONIN13  (via drill 0.61)
  Top 0.254: v72.58,56.69 72.58,58.06 72.69,58.18 72.69,59.09 v72.01,59.78
  Bottom 0.254: v72.58,56.69 74.07,55.21 77.04,55.21 78.07,54.18 78.07,53.26 78.64,52.81 79.21,52.81 84.58,47.55 84.58,46.86 87.33,44.01 IC1.12 | v72.01,59.78 70.98,60.81 70.98,68.58 69.49,70.07 OK4.2
DARLINGTONIN14  (via drill 0.61)
  Top 0.254: v88.35,51.44 88.01,51.09 87.33,51.09 85.72,49.49 85.72,48.58 87.33,46.98 87.33,46.52 IC1.13 | v70.75,72.12 70.75,69.95 68.58,67.78 66.75,67.78 64.47,70.07 OK4.4
  Bottom 0.254: v88.35,51.44 85.72,51.44 84.58,52.58 84.58,56.35 83.55,57.38 83.44,57.38 80.35,60.47 78.64,60.47 78.07,61.04 78.07,61.84 77.04,62.87 74.87,62.87 73.72,64.01 73.72,66.98 70.75,69.95 v70.75,72.12
DARLINGTONIN15  (via drill 0.61)
  Top 0.254: v69.15,64.24 68.47,64.24 66.06,66.64 62.87,66.64 59.44,70.07 OK4.6
  Bottom 0.254: v69.15,64.24 70.52,62.87 70.52,58.52 71.44,57.61 77.27,57.61 78.07,56.81 78.07,56.01 78.75,55.32 80.35,55.32 86.64,49.03 87.33,49.03 IC1.14
DARLINGTONIN16  (via drill 0.61)
  Top 0.254: v75.21,46.86 77.27,48.92 79.67,48.92 IC1.15 | v73.95,45.61 73.27,45.61 72.92,45.26 57.95,45.26 v55.89,47.32 | v54.41,48.35 54.41,48.58 53.15,49.84 53.15,60.12 51.55,61.72 51.55,64.69 48.46,67.78 43.09,67.78 41.83,69.04 41.83,71.09 42.98,72.24 52.12,72.24 OK4.8
  Bottom 0.254: v73.95,45.61 v75.21,46.86 | v55.89,47.32 55.44,47.32 v54.41,48.35
DARLINGTONIN17  (via drill 0.61)
  Top 0.254: OK5.2 66.29,80.12 67.78,78.64 67.78,72.01 68.24,71.55 v68.24,68.69 | v69.84,52.58 v69.84,55.21 | v77.38,39.89 81.72,39.89 86.75,34.86 93.73,34.86 95.33,33.26 95.33,18.52 92.81,16 IC2.28
  Bottom 0.254: v68.24,68.69 68.24,58.86 69.84,57.26 v69.84,55.21 | v69.84,52.58 72.58,49.84 72.58,44.69 v77.38,39.89
DARLINGTONIN18  (via drill 0.61)
  Top 0.254: v65.38,80.12 v61.84,80.12 | v85.15,73.27 85.15,66.64 86.3,65.49 88.58,65.49 90.64,67.55 93.84,67.55 94.87,66.52 94.87,56.46 93.27,54.86 91.55,54.86 90.98,54.29 90.98,48.58 92.01,47.55 93.84,47.55 94.41,48.12 94.41,49.84 95.78,51.21 96.58,51.21 98.64,49.15 98.64,17.6 100.24,16 IC2.1
  Bottom 0.254: v61.84,80.12 61.27,80.7 61.27,82.3 OK5.4 | v65.38,80.12 72.35,80.12 72.81,79.67 73.95,79.67 78.41,75.21 80.81,75.21 81.95,74.07 81.95,73.15 82.75,72.35 v85.15,73.27
DARLINGTONIN19  (via drill 0.61)
  Top 0.254: OK5.6 57.26,82.3 60.58,78.98 v66.18,78.98 | v71.55,78.98 72.01,78.98 72.92,79.9 74.98,79.9 v75.78,80.7 | v82.41,81.72 82.41,81.04 v83.33,80.12 | v94.64,82.53 94.64,81.95 96.81,79.78 v96.81,77.38
  Bottom 0.254: v71.55,78.98 v66.18,78.98 | v75.78,80.7 81.38,80.7 v82.41,81.72 | v83.33,80.12 86.18,80.12 86.3,80.24 89.04,80.24 91.67,82.87 94.3,82.87 v94.64,82.53 | v96.81,77.38 96.81,64.58 98.64,62.64 98.64,20.23 IC2.2
DARLINGTONIN20  (via drill 0.61)
  Top 0.254: v51.09,77.72 51.09,82.3 OK5.8 | v52.12,68.01 52.12,66.06 55.78,62.41 55.78,58.98 v62.18,52.58 | v62.29,36.46 62.29,33.95 v64.47,31.77 | v84.92,14.86 91.1,14.86 91.44,14.52 100.93,14.52 102.07,15.66 102.07,19.32 100.36,21.03 IC2.3
  Bottom 0.254: v51.09,77.72 51.09,76.12 52.12,75.09 v52.12,68.01 | v62.18,52.58 63.32,51.44 63.32,37.49 v62.29,36.46 | v64.47,31.77 69.72,31.77 71.89,29.6 71.89,29.38 79.1,22.17 80.81,22.17 81.5,21.37 81.5,18.06 v84.92,14.86
DARLINGTONIN21  (via drill 0.61)
  Top 0.254: v95.33,84.24 95.67,83.78 95.67,81.61 97.04,80.24 98.75,80.24 99.78,79.21 IC3.11 | v78.07,90.53 76.35,90.53 v73.5,93.38
  Bottom 0.254: v95.33,84.24 94.87,84.24 93.27,85.84 91.67,85.84 90.41,87.1 89.72,87.1 88.47,85.84 85.95,85.84 81.27,90.53 v78.07,90.53 | v73.5,93.38 69.49,93.38 69.27,93.15 67.32,93.15 66.29,94.18 OK6.2
DARLINGTONIN22  (via drill 0.61)
  Top 0.254: v62.98,92.47 OK6.4
  Bottom 0.254: v62.98,92.47 74.52,92.47 77.84,95.78 96.58,95.78 97.95,94.41 97.95,93.73 98.87,92.81 99.56,92.81 100.24,92.13 100.24,88.92 98.64,87.33 98.64,83.44 100.24,81.84 IC3.12
DARLINGTONIN23  (via drill 0.61)
  Top 0.254: v60.12,89.27 v60.12,91.55 | v65.49,58.41 65.49,54.52 v63.78,52.81 | v65.04,34.98 68.58,31.43 v68.58,27.89 | v75.78,22.97 79.21,19.55 84.24,19.55 86.75,17.03 89.61,17.03 91.67,14.97 93.84,14.97 v97.16,18.29 | v98.3,82.53 98.53,82.53 IC3.13
  Bottom 0.254: v60.12,91.55 59.89,91.55 57.26,94.18 56.24,94.18 OK6.6 | v60.12,89.27 62.75,86.64 62.75,72.01 63.32,71.44 63.32,65.04 65.49,62.87 v65.49,58.41 | v63.78,52.81 63.78,36.23 v65.04,34.98 | v68.58,27.89 68.58,25.26 70.87,22.97 v75.78,22.97 | v97.16,18.29 97.16,30.18 98.18,30.98 98.18,62.41 96.36,64.35 96.36,76.47 95.9,76.92 95.9,77.84 97.38,79.44 97.38,81.61 v98.3,82.53
DARLINGTONIN24  (via drill 0.61)
  Top 0.254: IC3.14 97.16,86.87 v95.33,88.7 | v61.38,91.55 60.47,92.47 52.81,92.47 51.09,94.18 OK6.8
  Bottom 0.254: v95.33,88.7 92.58,91.44 92.58,92.13 91.67,93.04 90.98,93.04 90.07,93.95 90.07,94.64 89.38,95.33 78.07,95.33 74.3,91.55 v61.38,91.55
DARLINGTONOUT1  (via drill 0.61)
  Top 0.305: v24,49.61 v24,44.81
  Bottom 0.305: v24,44.81 24,42.29 34.86,31.32 34.86,29.49 35.89,28.46 43.55,28.46 46.06,25.95 46.41,25.95 IC5.2 | v24,49.61 24,53.84 22.97,54.86 22.97,61.38 21.37,62.98 JP1.2
DARLINGTONOUT2  (via drill 0.61)
  Top 0.305: v23.09,36.23 23.09,41.83 20.46,44.46 20.46,62.18 20.12,62.52 20.12,64.35 21.26,65.49 JP1.4
  Bottom 0.305: v23.09,36.23 30.75,28.46 32.12,28.46 33.72,26.75 33.72,25.95 IC5.7
DARLINGTONOUT3  (via drill 0.61)
  Top 0.305: v21.83,27.66 21.83,28.23 19.55,30.52 v19.55,43.2
  Bottom 0.305: v21.83,27.66 31.2,18.29 IC5.9 | v19.55,43.2 19.55,53.15 18.17,54.52 18.17,65.72 20.46,68.01 21.26,68.01 JP1.6
DARLINGTONOUT4  (via drill 0.61)
  Top 0.305: v28.57,45.03 v28.57,26.4
  Bottom 0.305: IC5.16 48.69,18.29 45.61,21.49 33.6,21.49 v28.57,26.4 | v28.57,45.03 28.57,54.75 28,55.32 28,60.47 24.12,64.35 23.43,64.35 22.52,65.27 22.52,69.38 21.37,70.52 JP1.8
DARLINGTONOUT5  (via drill 0.61)
  Top 0.305: v45.03,47.43 45.03,41.49 46.41,40.12 46.41,37.95 IC6.2 | v41.95,53.95 40.35,53.95 39.43,54.86 39.43,56.24 38.86,56.81 37.49,56.81 36.92,57.38 36.92,58.75 33.83,61.84 33.83,64.35 25.03,73.15 25.03,73.61 24.12,74.52 23.43,74.52 22.52,75.44 22.52,76.12 21.83,76.81 20.8,76.81 20.12,76.12 20.12,74.3 21.26,73.15 JP1.10
  Bottom 0.305: v45.03,47.43 45.03,50.86 v41.95,53.95
DARLINGTONOUT6  (via drill 0.61)
  Top 0.305: v20.12,66.41 20.12,68.47 21.14,69.49 21.83,69.49 22.52,70.18 22.52,74.52 21.37,75.67 JP1.12
  Bottom 0.305: v20.12,66.41 20.12,62.52 20.46,62.18 20.46,48.35 24.92,45.49 24.92,43.78 29.83,38.98 29.83,37.15 30.86,36.12 31.66,36.12 33.38,37.83 33.72,37.83 IC6.7
DARLINGTONOUT7  (via drill 0.61)
  Top 0.305: v19.55,69.72 19.55,76.47 21.26,78.18 JP1.14
  Bottom 0.305: v19.55,69.72 19.09,69.72 10.52,61.15 10.52,45.26 11.77,44.01 16.23,44.01 21.95,38.06 22.52,38.06 30.29,30.29 31.2,30.29 IC6.9
DARLINGTONOUT8  (via drill 0.61)
  Top 0.305: v49.03,35.66 50.98,37.6 50.98,43.66 55.66,48.35 55.66,58.29 52.12,61.84 52.12,64.81 48.58,68.35 44.58,68.35 v44.23,68.69
  Bottom 0.305: v49.03,35.66 49.03,30.29 IC6.16 | v44.23,68.69 44.23,70.98 42.29,72.92 32.35,72.92 31.32,73.95 31.32,75.78 25.15,81.95 22.52,81.95 JP1.16
DARLINGTONOUT9  (via drill 0.61)
  Top 0.305: v47.43,39.55 48.58,39.55 50.06,41.03 50.06,44.35 46.52,47.89 46.52,49.72 IC7.2
  Bottom 0.305: v47.43,39.55 30.06,39.55 25.49,44.12 25.49,61.38 JP1.1
DARLINGTONOUT10
  Bottom 0.305: IC7.7 33.72,49.84 33.72,50.41 28.57,55.55 28.57,60.81 23.89,65.49 JP1.3
DARLINGTONOUT11
  Top 0.305: IC7.9 31.2,42.18 31.2,43.66 22.97,51.89 22.97,62.29 22.75,62.52 22.75,66.98 23.77,68.01 JP1.5
DARLINGTONOUT12  (via drill 0.61)
  Top 0.305: v33.6,47.66 32.35,48.92 32.35,51.78 28,56.12 28,66.41 23.89,70.52 JP1.7
  Bottom 0.305: v33.6,47.66 36.8,44.46 46.29,44.46 48.58,42.18 48.92,42.18 IC7.16
DARLINGTONOUT13
  Bottom 0.305: IC8.2 45.38,70.07 45.38,68.58 44.58,67.78 43.09,67.78 41.83,69.04 41.83,70.87 40.35,72.35 30.4,72.35 25.6,77.15 25.6,78.18 24.35,79.44 23.43,79.44 22.75,78.75 22.75,74.18 23.77,73.15 JP1.9
DARLINGTONOUT14  (via drill 0.61)
  Top 0.305: v27.77,71.78 23.89,75.67 JP1.11
  Bottom 0.305: v27.77,71.78 30.75,71.78 32.35,70.18 32.69,70.18 IC8.7
DARLINGTONOUT15
  Bottom 0.305: IC8.9 30.18,62.52 30.18,63.44 27.09,66.52 27.09,70.07 25.03,72.12 25.03,77.04 23.89,78.18 JP1.13
DARLINGTONOUT16
  Top 0.305: IC8.16 48.01,62.41 47.55,62.41 45.95,60.81 37.38,60.81 36.35,61.84 36.35,64.35 31.32,69.38 31.32,71.44 25.38,77.38 25.38,83.78 23.89,85.27 JP2.1
DARLINGTONOUT17  (via drill 0.61)
  Top 0.305: IC9.2 45.03,82.3 43.32,84.01 42.52,84.01 41.83,83.33 41.83,81.04 v39.89,79.1
  Bottom 0.305: v39.89,79.1 28.8,79.1 23.77,84.12 22.52,84.12 21.37,85.27 JP2.2
DARLINGTONOUT18
  Bottom 0.305: IC9.7 31.43,80.47 29.49,80.47 28.92,81.04 28.92,83.21 24.35,87.78 23.89,87.78 JP2.3
DARLINGTONOUT19
  Top 0.305: IC9.9 30.18,74.75 30.18,80.24 25.15,85.27 25.15,85.84 24.23,86.75 22.4,86.75 21.37,87.78 JP2.4
DARLINGTONOUT20  (via drill 0.61)
  Top 0.305: v35.43,80.01 32.12,80.01 31.43,80.81 v31.43,85.04
  Bottom 0.305: v35.43,80.01 42.29,80.01 47.55,74.75 48.01,74.75 IC9.16 | v31.43,85.04 31.43,88.01 30.86,88.47 29.03,88.47 27.2,90.41 JP2.5
DARLINGTONOUT21  (via drill 0.61)
  Top 0.305: v25.38,92.47 33.15,92.47 33.83,93.15 33.83,94.87 34.98,96.01 43.32,96.01 45.03,94.3 45.38,94.3 IC10.2
  Bottom 0.305: v25.38,92.47 25.03,92.47 24.23,91.78 22.52,91.78 21.37,90.53 JP2.6
DARLINGTONOUT22
  Top 0.305: IC10.7 32.69,94.3 32.35,94.3 30.63,96.01 26.86,96.01 23.89,93.04 JP2.7
DARLINGTONOUT23
  Top 0.305: JP2.8 22.52,91.9 24.23,91.9 29.26,86.64 30.18,86.64 IC10.9
DARLINGTONOUT24
  Bottom 0.305: JP2.9 25.72,95.44 32.35,88.47 33.38,88.47 33.95,87.78 33.95,85.61 34.75,84.7 46.75,84.7 IC10.16
FLIPPER_RGB1  (via drill 0.61)
  Top 0.254: v85.5,47.32 85.5,46.29 86.75,45.03 89.5,45.03 91.67,42.86 93.73,42.86 95.78,44.58 v95.78,49.84 | v94.53,53.03 94.53,53.61 98.3,57.38 v98.3,69.15 | v107.9,82.07 107.9,83.1 109.5,84.7 109.5,86.87 102.18,94.18 101.61,94.18 JP3.1
  Bottom 0.254: v85.5,47.32 79.78,53.03 79.78,53.84 IC4.28 | v95.78,49.84 94.53,51.44 v94.53,53.03 | v98.3,69.15 99.78,70.64 102.87,70.64 104.93,72.69 104.93,79.1 v107.9,82.07
FLIPPER_RGB2  (via drill 0.61)
  Top 0.254: v94.53,54.86 94.53,55.44 97.38,58.29 97.38,73.38 v98.3,74.3
  Bottom 0.254: v94.53,54.86 91.55,54.86 90.64,53.95 87.44,53.95 IC4.1 | v98.3,74.3 99.67,75.67 101.38,75.67 102.3,76.58 102.3,78.41 102.98,79.1 102.98,82.41 104.47,83.9 104.47,90.41 101.84,93.04 100.24,93.04 99.1,94.18 JP3.3
FLIPPER_RGB3
  Top 0.254: IC4.2 87.33,56.46 87.33,56.81 84.24,59.89 84.24,81.95 80.35,85.84 78.64,85.84 78.07,86.41 78.07,87.33 81.27,90.53 81.72,90.53 82.64,91.44 82.64,94.64 83.33,95.33 95.44,95.33 96.47,94.3 JP3.5
FLIPPER_RGB4  (via drill 0.61)
  Top 0.254: v76.69,66.75 76.12,67.78 76.12,75.21 79.1,78.18 80.81,78.18 82.07,79.44 v82.07,80.12 | v90.07,86.18 90.07,91.9 91.21,93.04 92.81,93.04 93.95,94.18 JP3.7
  Bottom 0.254: v76.69,66.75 78.07,64.92 78.07,63.55 78.64,62.98 80.35,62.98 84.35,58.98 87.33,58.98 IC4.3 | v82.07,80.12 82.98,81.04 85.95,81.04 86.3,80.7 88.35,80.7 90.98,83.33 90.98,85.27 v90.07,86.18
FLIPPER_RGB5
  Bottom 0.254: IC4.4 87.44,61.49 88.12,61.49 92.13,65.49 93.73,65.49 94.87,66.64 94.87,77.61 96.93,79.67 96.93,90.53 97.61,91.21 97.61,92.24 96.81,93.04 92.58,93.04 91.44,94.18 JP3.9
FLIPPER_RGB6  (via drill 0.61)
  Top 0.254: v82.87,73.5 83.33,73.04 83.33,67.78 82.75,67.21 82.75,55.66 83.33,55.09 88.24,55.09 89.04,55.89 89.04,61.95 87.44,63.55 87.44,64.01 IC4.5 | v85.61,75.78 85.61,77.04 86.75,78.18 88.47,78.18 89.04,78.75 89.04,82.3 88.01,83.33 86.3,83.33 85.72,83.9 85.72,87.67 87.9,89.84 v87.9,90.41
  Bottom 0.254: v82.87,73.5 83.33,73.5 v85.61,75.78 | v87.9,90.41 87.9,91.1 87.78,91.21 87.78,93.15 88.81,94.18 JP3.11
FLIPPER_RGB7  (via drill 0.61)
  Top 0.254: v98.3,76.35 97.38,75.44 97.38,74.18 93.84,70.64 92.13,70.64 90.98,69.49 90.98,68.69 88.92,66.64 87.44,66.64 IC4.6
  Bottom 0.254: v98.3,76.35 98.3,76.81 99.67,78.18 101.38,78.18 102.53,79.32 102.53,82.64 102.98,83.1 102.98,84.12 102.07,85.04 102.07,91.21 101.61,91.67 JP3.2
FLIPPER_RGB8  (via drill 0.61)
  Top 0.254: v98.3,79.32 98.3,77.61 93.84,73.15 92.13,73.15 90.98,72.01 90.98,71.21 90.41,70.64 89.95,70.64 88.47,69.15 87.44,69.15 IC4.7 | v102.07,83.44 102.07,88.7 99.1,91.67 JP3.4
  Bottom 0.254: v98.3,79.32 99.67,80.7 101.38,80.7 102.07,81.38 v102.07,83.44
FLIPPER_RGB9  (via drill 0.61)
  Top 0.254: v90.98,75.78 90.98,77.15 92.01,78.18 93.73,78.18 94.41,78.87 v94.41,80.24
  Bottom 0.254: v90.98,75.78 90.98,73.72 90.41,73.15 89.95,73.15 88.47,71.67 87.44,71.67 IC4.8 | v94.41,80.24 94.41,81.04 96.47,83.1 96.47,91.67 JP3.6
FLIPPER_RGB10
  Top 0.254: IC4.9 87.44,74.18 87.44,74.64 90.98,78.18 90.98,82.18 92.13,83.33 93.84,83.33 94.41,83.9 94.41,91.33 94.07,91.67 JP3.8
FLIPPER_RGB11
  Top 0.254: IC4.10 87.44,76.81 87.78,76.81 90.53,79.55 90.53,83.44 90.98,83.9 90.98,91.21 91.44,91.67 JP3.10
FLIPPER_RGB12  (via drill 0.61)
  Top 0.254: v85.95,89.84 85.95,89.27 84.81,88.12 84.81,82.18 87.33,79.67 87.33,79.32 IC4.11
  Bottom 0.254: v85.95,89.84 87.21,89.84 87.55,89.5 88.24,89.5 88.81,90.07 88.81,91.67 JP3.12
FLIPPER_RGB13
  Top 0.254: JP3.13 87.55,93.04 87.55,91.33 86.98,90.75 86.98,89.61 85.27,87.9 85.27,83.67 87.1,81.84 87.33,81.84 IC4.12
FLIPPER_RGB14  (via drill 0.61)
  Top 0.254: v82.64,87.9 82.64,88.92 84.92,91.21 84.92,93.15 83.9,94.18 JP3.15
  Bottom 0.254: v82.64,87.9 86.18,84.35 87.33,84.35 IC4.13
FLIPPER_RGB15
  Bottom 0.254: IC4.14 87.1,86.87 82.41,91.55 82.41,93.15 81.38,94.18 JP3.17
FLIPPER_RGB16
  Top 0.254: IC4.15 82.87,86.87 85.04,89.04 85.04,90.41 86.3,91.67 JP3.14
GND  (via drill 0.61)
  Top 0.457: FRDM1.GND2 11.66,57.95 11.2,57.95 6.86,62.29 5.37,62.29 JP8.2 | OK15.2 14.4,70.41 14.4,71.67 12,74.07 R16.1 11.77,74.18 9.26,76.69 | 9.26,76.69 1.83,76.69 R36.1 | JP5.26 11.2,2.86 11.2,3.09 9.6,4.69 9.6,30.75 14.74,38.18 14.74,38.75 T1.E | C4.1 77.72,69.15 79.67,69.15 IC4.22 79.9,68.92 79.9,68.69 82.18,66.41 82.18,52.01 v84.12,50.06 | C11.- 73.15,78.52 74.98,78.52 77.15,80.7 77.15,84.24 R5.2 | T2.C 111.56,13.37 111.56,11.2 109.5,9.14 C8.- | IC11.1 122.99,10.29 122.99,8.69 119.44,5.14 112.58,5.14 C7.2 112.36,5.03 110.76,5.03 109.61,3.89 C5.- 109.39,3.77 108.13,2.52 106.53,2.52 105.73,3.31 105.73,4.23 109.39,7.89 109.39,9.03 C8.- | JP7.6 60.92,1.6 51.55,1.6 50.41,2.74 49.49,2.74 JP6.4 | C2.1 90.75,31.32 92.7,31.32 IC2.22 | C6.1 75.44,30.06 76.58,30.06 77.72,31.2 C1.1 | IC1.22 79.67,31.32 77.84,31.32 C1.1 | C10.+ 75.21,33.95 77.72,31.43 C1.1 | v107.56,10.86 109.27,9.14 C8.- | v13.26,92.01 12,90.75 11.66,90.75 9.37,88.47 9.37,76.81 9.26,76.69
  Bottom 0.457: FRDM1.GND0 28.12,9.72 25.72,9.72 FRDM1.GND1 25.72,9.83 24.46,11.09 24.46,12.92 24,13.37 12.12,13.37 11.77,13.03 11.77,8.8 12.57,8 12.57,4.92 11.32,3.66 11.32,2.86 JP5.26 | 14.74,38.86 T1.E 13.14,40.8 8.91,40.8 T3.E 7.43,38.98 7.43,52.46 5.37,54.52 JP8.2 6.86,62.41 14.4,69.95 14.4,70.29 OK15.2 | IC3.22 92.7,69.15 89.95,69.15 C3.1 89.72,69.15 88.7,70.18 86.18,70.18 85.15,69.15 79.78,69.15 IC4.22 | 74.3,89.04 73.15,90.18 IC12.1 73.04,90.3 60.01,90.3 59.32,90.98 30.98,90.98 25.38,96.93 20.8,96.93 17.37,93.27 14.52,93.27 v13.26,92.01 | 74.3,89.04 77.15,86.18 77.15,84.35 R5.2 77.38,84.24 78.41,83.21 88.47,83.21 89.5,84.24 89.84,84.24 R4.2 | 74.3,89.04 77.15,91.9 C12.2 | C4.1 77.72,70.07 73.15,74.64 C11.- | 90.07,41.83 88.47,40.23 86.3,40.23 81.5,45.03 78.98,45.03 77.61,46.41 77.04,46.41 R2.2 | 90.07,41.83 90.07,46.41 R3.2 89.84,46.41 88.58,47.66 86.53,47.66 v84.12,50.06 | IC1.22 79.78,31.32 80.81,32.35 88.58,32.35 89.61,31.32 90.64,31.32 C2.1 90.75,31.09 90.75,15.66 91.55,14.86 93.04,14.86 95.21,12.69 95.21,11.66 | 95.21,11.66 90.98,7.43 76.81,7.43 70.98,1.6 63.89,1.6 62.75,2.74 62.18,2.74 JP7.6 | 90.07,41.83 91.9,40.01 93.84,40.01 94.98,38.86 94.98,33.49 92.81,31.32 IC2.22 | v107.56,10.86 96.01,10.86 95.21,11.66
  pour Bottom: 0.11,99.56 159.45,99.56 159.45,0.11 0.11,0.23
GND1  (2 unrouted)
  Top 0.254: IC10.12 U$3.P$2
  Top 2.032: IC5.12 39.05,18.41 39.05,25.72 IC5.5 39.05,26.67 39.05,30.16 IC6.12 39.05,31.11 39.05,37.15 IC6.5 39.05,38.1 39.05,41.91 IC7.12 39.05,42.86 39.05,49.53 IC7.5 | 38.1,65.09 38.1,69.85 IC8.5 38.1,70.8 38.1,74.61 IC9.12 38.1,75.56 38.1,82.23 IC9.5 | 38.1,65.09 38.1,62.55 IC8.12 | IC9.4 40.32,82.55 40.32,83.82 40.64,84.14 40.64,86.36 IC10.13 40.01,87.31 39.69,87.63 39.69,93.34 40.32,93.98 IC10.4 | 38.1,65.09 49.24,65.09 50.18,64.15 50.18,60.62 51.7,59.28 51.66,53.68 50.8,52.7 43.5,52.7 41.27,50.48 41.27,49.85 IC7.4
  Bottom 2.032: IC6.12 39.05,30.16 41.27,30.16 IC6.13 | IC5.12 39.05,18.41 41.27,18.41 IC5.13 | IC5.5 39.05,26.04 41.27,26.04 IC5.4 | IC7.5 39.05,49.85 41.27,49.85 IC7.4 | IC6.5 39.05,37.78 41.27,37.78 IC6.4 | IC7.12 39.05,42.23 41.27,42.23 IC7.13 | IC10.12 38.1,86.68 40.32,86.68 IC10.13 | IC9.5 38.1,82.23 40.32,82.23 IC9.4 | IC9.12 38.1,74.61 40.32,74.61 IC9.13 | IC8.12 38.1,62.55 40.32,62.55 IC8.13 | IC8.5 38.1,70.17 40.32,70.17 IC8.4 | IC10.5 38.1,94.3 40.32,94.3 IC10.4 40.32,95.25 42.55,97.47 101.98,97.59 105.16,94.53 106.64,92.24 110.19,92.24 U$4.P$1 U$2.P$2
GND2  (via drill 0.61)
  Top 0.254: T4.E 15.32,91.9 12.92,89.5 12,89.5 R46.1 11.89,89.38 11.89,88.24 10.52,86.87 v10.52,76.81 | v6.17,36.35 6.17,35.55 7.54,34.18 7.54,33.83 T6.E | v33.38,84.58 36.92,84.58 U$3.P$1
  Bottom 0.254: T6.E 7.66,33.72 7.66,32.23 10.86,29.03 OK13.2 | v10.52,76.81 10.52,72.47 2.97,64.92 2.97,48.12 6.17,44.92 v6.17,36.35 | T4.E 18.29,89.27 24.8,89.27 30.06,84.01 32.69,84.01 v33.38,84.58
GND3  (via drill 0.61)
  Top 1.524: 138.94,96.01 R32.1 138.94,96.77 | 138.94,95.38 138.94,96.01 | 138.94,96.01 139.06,96.01
  Top 1.575: R34.1 154.53,80.01 157.05,82.53 Q12C.3 156.13,82.64 152.93,85.84 v152.93,86.87 | R32.1 138.99,97.95 138.94,96.77 | R7.1 135.79,2.97 137.41,3.68 139.22,2.74 142.42,2.74 Q7A.3 | R14.1 138.99,5.26 137.41,5.26 | R24.1 135.9,10.86 137.87,13.72 | R26.1 138.53,14.74 137.41,14.48 | R20.1 133.62,20.34 135.25,20.35 | R19.1 136.25,23.55 135,19.31 | R22.1 135.19,29.73 | R9.1 136.13,33.03 135.18,33.03 | R13.1 133.62,39.66 135.14,44.81 | R11.1 136.47,42.98 135.12,42.97 | R17.1 133.62,48.58 135.09,48.59 | R15.1 136.47,51.78 135.07,51.77 | R25.1 133.62,57.38 135.04,59.67 | R23.1 136.13,60.81 135.02,60.8 | R27.1 133.62,69.84 134.99,69.84 | R29.1 136.13,70.07 134.97,70.06 | R28.1 133.39,75.21 134.94,78.42 | R30.1 136.13,78.64 134.93,78.63 | R31.1 133.27,84.47 134.78,86.31 | R35.1 136.13,87.67 134.88,87.66 | 134.53,91.39 133.39,90.98 135.33,90.65 | 137.99,4.34 133.27,5.49 Q7B.3 | 137.41,13.72 Q7D.3 | Q8A.3 138.88,21.03 137.27,21.03 135.24,21.02 | Q8B.3 133.27,22.86 135.23,22.87 | Q8C.3 138.88,30.52 137.16,30.52 135.19,30.51 | Q8D.3 131.33,32.35 133.16,32.35 135.18,32.36 | Q9B.3 131.33,42.18 133.16,42.18 135.13,42.19 | 135.14,40.45 137.16,40.46 138.88,40.46 Q9A.3 139.45,42.04 141.6,44.2 144.65,44.2 146.05,44.96 148.08,44.96 v148.34,46.86 | Q9D.3 131.33,51.09 133.04,51.09 135.08,51.1 | Q9C.3 138.88,49.38 137.05,49.38 135.09,49.37 | Q10C.3 131.33,60.01 133.04,60.01 135.03,60.02 | Q10B.3 137.05,58.29 135.04,58.28 | Q10D.3 131.33,69.38 132.93,69.38 134.98,69.39 | Q11B.3 138.88,67.67 136.93,67.67 134.99,67.66 | Q11A.3 132.93,77.72 134.93,77.73 | Q11C.3 138.88,76.12 136.93,76.12 134.94,76.11 | Q11D.3 132.93,86.87 134.88,86.88
  Top 1.575: Q12D.3 138.88,85.15 136.93,85.15 134.89,85.14 | Q12B.3 134.07,97.16 134.07,96.93 134.76,96.24 R33.1 | 137.41,12.23 141.5,12.23 Q7C.3 | Q12A.3 142.19,95.56 140.93,95.56 138.94,95.38 | Q10A.3 156.59,44.01 154.08,41.49 R21.1 | U$4.P$2 116.04,96.03
  Top 2.032: 137.99,4.34 137.41,3.68 | 113.73,90.75 116.04,96.03 116.13,96.24
  Top 4.115: 134.53,91.39 134.75,90.93 138.94,95.38 | R33.1 135.33,90.65 | 134.87,88.01 134.88,87.66 134.88,86.88 134.89,85.14 134.78,86.31 | 134.93,78.63 134.93,77.73 134.94,76.11 134.94,78.42 | 134.97,70.06 134.98,69.39 134.99,67.66 134.99,69.84 | 135.02,60.8 135.03,60.02 135.04,58.28 135.04,59.67 | 135.07,51.77 135.08,51.1 | 135.09,49.37 135.09,48.59 | 135.12,42.97 135.13,42.19 135.14,40.45 135.14,44.81 | 135.18,33.03 135.18,32.36 135.19,30.51 135.19,29.73 | 135,19.31 135.23,22.87 135.24,21.02 135.25,20.35 135.25,18.92 | 137.41,14.48 137.41,13.72 137.41,12.23 137.87,13.72 | 137.41,5.26 137.99,4.34
  Top 5.309: 134.53,91.39 124.5,91.39 120.47,90.75 113.73,90.75 | 135.33,90.65 134.87,88.01 | 134.78,86.31 134.93,78.63 | 134.94,78.42 134.97,70.06 | 134.99,69.84 135.02,60.8 | 135.04,59.67 135.07,51.77 | 135.08,51.1 135.09,49.37 | 135.09,48.59 135.12,42.97 | 135.14,44.81 135.18,33.03 | 135.19,29.73 135,19.31 | 135.25,18.92 137.41,14.48 | 137.87,13.72 137.99,4.34
  Bottom 1.575: v152.93,86.87 152.59,86.87 149.96,89.5 138.07,89.5 136.25,87.67 R35.1 | v148.34,46.86 149.73,46.86 R21.1
HICURRENT5V
  Top 2.032: 18.86,96.71 19.79,97.66 105.39,97.66 JP4.4 | 18.86,96.71 18.86,84.92 20.56,83.06 22.62,83.06 23.89,81.61 JP1.15 | 18.86,96.71 U$1.P$1
KEYS1
  Top 0.254: FRDM1.A4 45.95,9.6 41.72,5.37 JP5.1
KEYS2
  Top 0.254: FRDM1.A3 43.43,8.57 40.69,5.83 40.69,3.89 JP5.2
KEYS3
  Top 0.254: FRDM1.A2 40.8,9.6 40.8,6.86 39.32,5.37 JP5.3
KEYS4
  Top 0.254: FRDM1.A1 38.29,9.6 38.29,5.94 38.06,5.71 38.06,4 39.2,2.86 JP5.4
KEYS5
  Bottom 0.254: FRDM1.PTE30 48.46,12.12 47.78,12.12 46.41,10.74 45.03,10.74 44.69,10.4 44.69,8.91 42.41,6.74 38.18,6.74 36.8,5.37 JP5.5
KEYS6  (via drill 0.61)
  Top 0.254: v37.15,22.63 37.38,22.97 37.38,26.98 35.32,29.03 35.32,50.41 30.75,54.98 30.75,55.32 FRDM1.PTC11
  Bottom 0.254: v37.15,22.63 37.38,22.29 47.32,22.29 50.06,19.32 50.06,11.77 49.03,10.74 47.66,10.74 47.09,10.17 47.09,8.8 42.18,3.89 37.83,3.89 36.8,2.86 JP5.6
KEYS7
  Top 0.254: FRDM1.PTE5 31.89,12.12 34.06,9.94 34.06,5.37 JP5.7
KEYS8
  Top 0.254: FRDM1.PTE4 28.46,12.12 29.38,11.32 29.95,10.86 31.55,10.86 33.03,9.37 33.03,3.89 34.06,2.86 JP5.8
KEYS9
  Bottom 0.254: FRDM1.PTE3 25.72,12.12 26.29,12.12 27.66,10.74 29.03,10.74 29.6,10.17 29.6,7.32 31.55,5.37 JP5.9
KEYS10
  Bottom 0.254: FRDM1.PTE2 23.2,12.12 23.2,11.54 24.57,10.17 24.57,8.8 26.86,6.51 29.49,6.51 30.52,5.49 30.52,3.89 31.55,2.86 JP5.10
KEYS11
  Bottom 0.254: FRDM1.PTB11 20.57,11.54 22.06,10.06 22.06,8.8 24.35,6.51 24.46,6.51 25.38,5.6 25.38,4.92 26.06,4.23 28,4.23 29.03,5.26 JP5.11
KEYS12  (via drill 0.61)
  Top 0.254: v19.55,6.74 19.43,6.86 19.43,10.17 18.06,11.54 18.06,12.12 FRDM1.PTB10
  Bottom 0.254: v19.55,6.74 19.55,6.29 20.34,5.49 20.34,4.8 21.26,3.89 21.95,3.89 22.86,2.97 22.86,2.29 23.55,1.6 27.89,1.6 JP5.12
KEYS13
  Top 0.254: FRDM1.PTB9 15.54,12.23 15.54,13.49 19.09,17.03 21.6,17.03 24.46,12.92 24.46,11.32 24.8,10.97 26.52,10.97 26.98,10.52 26.98,5.83 JP5.13
KEYS14
  Bottom 0.254: FRDM1.PTB8 13.03,12.12 13.03,11.54 14.4,10.17 14.4,8.8 15.54,7.66 20.69,7.66 22.86,5.49 22.86,4.92 23.89,3.89 25.49,3.89 26.52,2.86 JP5.14
KEYS15  (via drill 0.61)
  Top 0.254: v26.86,45.61 26.86,20.57 v26.52,19.66 | v21.14,16.12 21.14,13.6 21.95,12.8 21.95,11.32 22.29,10.97 23.89,10.97 24.46,10.4 24.46,5.94 24,5.37 JP5.15
  Bottom 0.254: v26.86,45.61 26.86,55.32 FRDM1.PTC12 | v21.14,16.12 v26.52,19.66
KEYS16
  Top 0.254: FRDM1.PTC13 24.46,55.32 24.46,51.09 32.23,43.32 32.23,23.32 29.6,20.69 29.6,15.2 34.75,10.06 34.75,6.4 35.32,5.83 35.32,2.4 34.52,1.6 25.15,1.6 24,2.74 JP5.16
KEYS17  (via drill 0.61)
  Top 0.254: FRDM1.PTC16 21.83,43.89 24.12,41.83 24.12,28.69 25.6,27.32 25.6,16.57 v26.06,16.12 | JP5.17 21.72,5.71 21.83,5.94 21.83,10.4 21.37,10.86 19.77,10.86 19.32,11.32 v19.32,14.97
  Bottom 0.254: v19.32,14.97 24.92,14.97 v26.06,16.12
KEYS18  (via drill 0.61)
  Top 0.254: v22.17,29.95 22.17,41.83 19.32,44.69 19.32,55.32 FRDM1.PTC17
  Bottom 0.254: v22.17,29.95 22.17,29.38 30.29,21.26 30.86,21.26 32.69,19.43 32.69,14.63 33.03,14.29 33.03,2.63 31.55,1.14 23.09,1.14 21.49,2.74 JP5.18
KEYS19  (via drill 0.61)
  Top 0.254: v18.63,44.12 18.63,17.26 14.4,13.03 14.4,11.32 14.97,10.74 16.34,10.74 16.92,10.17 16.92,7.32 18.86,5.37 JP5.19
  Bottom 0.254: v18.63,44.12 16.8,45.95 16.8,55.32 FRDM1.PTA16
KEYS20
  Top 0.254: FRDM1.PTA17 14.29,55.32 14.29,45.95 15.43,44.81 15.43,41.26 14.74,40.58 14.29,40.58 13.26,39.55 13.26,37.26 9.03,31.2 9.03,3.43 10.86,1.6 17.72,1.6 18.86,2.74 JP5.20
KEYS21  (via drill 0.61)
  Top 0.254: v21.26,40.8 21.26,29.49 25.15,25.6 25.15,14.63 26.98,13.03 26.98,11.43 27.66,10.74 29.03,10.74 29.6,10.17 29.6,8 28.57,6.74 27.66,5.83 27.66,4.8 27.09,4.23 17.49,4.23 JP5.21
  Bottom 0.254: v21.26,40.8 20.34,40.8 16.69,44.58 12,44.58 11.32,45.26 11.32,46.63 11.66,46.86 11.66,55.32 FRDM1.PTE31
KEYS22  (via drill 0.61)
  Top 0.254: v15.89,36.01 15.89,19.09 10.97,14.17 10.97,7.32 12.69,5.6 12.69,4.92 13.72,3.89 15.32,3.89 16.34,2.86 JP5.22
  Bottom 0.254: v15.89,36.01 15.89,39.78 15.77,40.35 14.63,41.49 11.43,41.49 9.94,43.2 9.94,50.75 6.63,54.06 6.63,55.32 FRDM1.PTD6
KEYS23  (via drill 0.61)
  Top 0.254: v14.4,42.52 13.03,44.01 11.77,44.01 4.12,51.66 4.12,55.32 FRDM1.PTD7 | v16.8,40.8 16.8,19.32 11.43,13.95 11.43,7.77 13.83,5.37 JP5.23
  Bottom 0.254: v16.8,40.8 v14.4,42.52
KEYS24
  Top 0.254: FRDM1.D15 4.12,57.84 4.8,57.84 6.17,56.46 15.09,56.46 15.66,55.89 15.66,45.49 15.89,45.26 15.89,37.6 13.26,34.75 13.26,17.14 10.17,14.06 10.17,4.92 11.2,3.89 12.8,3.89 13.83,2.86 JP5.24
KNOCKER+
